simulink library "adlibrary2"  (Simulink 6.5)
undefined symbols (not defined in the file or in its folder): adlibrary2, ADM, DDRII, II, no_bitstream, SRAM, SX, XP, XRC
libraries: xbsIndex_r4 x360, adlibrary2 x9, adlibrary2_d2sram_0 x5, adlibrary2_ddr2dram_1 x4, adlibrary2_ddr_xpi0 x4, adlibrary2_ddr_xpl x3, adlibrary2_xpl32 x1, adlibrary2_xpl64 x1, adlibrary2_zbt64 x1, adlibrary2_zbt4_0 x1, adlibrary2_zbt4_1 x1, adlibrary2_zbt4_2 x1
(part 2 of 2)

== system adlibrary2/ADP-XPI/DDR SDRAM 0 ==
  cache_data_in : Inport
  cache_addr : Inport  Port=2
  cache_write : Inport  Port=3
  ddr_page : Inport  Port=4
  ddr_addr : Inport  Port=5
  ddr_read : Inport  Port=6
  ddr_write : Inport  Port=7
  Assert{1..7,9..10} (9 alike) : xbsIndex_r4/Assert  assert_type=off  type_source=Explicitly  arith_type="Signed  (2's comp)"  n_bits=16  bin_pt=14  assert_rate=on  rate_source=Explicitly  period=ad_get_simulink_period  output_port=on  block_type=assert
  Configurable Subsystem : Subsystem  Tag=configX  BlockChoice=DDR SDRAM 64bit Simulation  mask{memsize=memsize}
      mask prompts: memsize "Simulation Ram Size (Mb)"
  cache_data_out : Outport
  ddr_busy : Outport  Port=2
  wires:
  Assert10/1 -> ddr_busy/1
  Assert9/1 -> cache_data_out/1
  Assert6/1 -> Configurable Subsystem/6(ddr_read)
  Assert5/1 -> Configurable Subsystem/5(ddr_addr)
  Assert4/1 -> Configurable Subsystem/4(ddr_page)
  Assert3/1 -> Configurable Subsystem/3(cache_write)
  Assert2/1 -> Configurable Subsystem/2(cache_addr)
  Assert1/1 -> Configurable Subsystem/1(cache_data_in)
  ddr_write/1 -> Assert7/1
  ddr_read/1 -> Assert6/1
  ddr_addr/1 -> Assert5/1
  ddr_page/1 -> Assert4/1
  cache_write/1 -> Assert3/1
  cache_addr/1 -> Assert2/1
  cache_data_in/1 -> Assert1/1
  Configurable Subsystem/1(cache_data_out) -> Assert9/1
  Configurable Subsystem/2(ddr_busy) -> Assert10/1
  Assert7/1 -> Configurable Subsystem/7(ddr_write)

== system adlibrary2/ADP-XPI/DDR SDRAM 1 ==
  cache_data_in : Inport
  cache_addr : Inport  Port=2
  cache_write : Inport  Port=3
  ddr_page : Inport  Port=4
  ddr_addr : Inport  Port=5
  ddr_read : Inport  Port=6
  ddr_write : Inport  Port=7
  Assert{1..7,9..10} (9 alike) : xbsIndex_r4/Assert  assert_type=off  type_source=Explicitly  arith_type="Signed  (2's comp)"  n_bits=16  bin_pt=14  assert_rate=on  rate_source=Explicitly  period=ad_get_simulink_period  output_port=on  block_type=assert
  Configurable Subsystem : Subsystem  Tag=configX  BlockChoice=DDR SDRAM 64bit Simulation  mask{memsize=memsize}
      mask prompts: memsize "Simulation Ram Size (Mb)"
  cache_data_out : Outport
  ddr_busy : Outport  Port=2
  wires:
  Assert7/1 -> Configurable Subsystem/7(ddr_write)
  Configurable Subsystem/2(ddr_busy) -> Assert10/1
  Configurable Subsystem/1(cache_data_out) -> Assert9/1
  cache_data_in/1 -> Assert1/1
  cache_addr/1 -> Assert2/1
  cache_write/1 -> Assert3/1
  ddr_page/1 -> Assert4/1
  ddr_addr/1 -> Assert5/1
  ddr_read/1 -> Assert6/1
  ddr_write/1 -> Assert7/1
  Assert1/1 -> Configurable Subsystem/1(cache_data_in)
  Assert2/1 -> Configurable Subsystem/2(cache_addr)
  Assert3/1 -> Configurable Subsystem/3(cache_write)
  Assert4/1 -> Configurable Subsystem/4(ddr_page)
  Assert5/1 -> Configurable Subsystem/5(ddr_addr)
  Assert6/1 -> Configurable Subsystem/6(ddr_read)
  Assert9/1 -> cache_data_out/1
  Assert10/1 -> ddr_busy/1

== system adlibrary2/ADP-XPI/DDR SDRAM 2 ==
  cache_data_in : Inport
  cache_addr : Inport  Port=2
  cache_write : Inport  Port=3
  ddr_page : Inport  Port=4
  ddr_addr : Inport  Port=5
  ddr_read : Inport  Port=6
  ddr_write : Inport  Port=7
  Assert{1..7,9..10} (9 alike) : xbsIndex_r4/Assert  assert_type=off  type_source=Explicitly  arith_type="Signed  (2's comp)"  n_bits=16  bin_pt=14  assert_rate=on  rate_source=Explicitly  period=ad_get_simulink_period  output_port=on  block_type=assert
  Configurable Subsystem : Subsystem  Tag=configX  BlockChoice=DDR SDRAM 64bit Simulation  mask{memsize=memsize}
      mask prompts: memsize "Simulation Ram Size (Mb)"
  cache_data_out : Outport
  ddr_busy : Outport  Port=2
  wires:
  Assert10/1 -> ddr_busy/1
  Assert9/1 -> cache_data_out/1
  Assert6/1 -> Configurable Subsystem/6(ddr_read)
  Assert5/1 -> Configurable Subsystem/5(ddr_addr)
  Assert4/1 -> Configurable Subsystem/4(ddr_page)
  Assert3/1 -> Configurable Subsystem/3(cache_write)
  Assert2/1 -> Configurable Subsystem/2(cache_addr)
  Assert1/1 -> Configurable Subsystem/1(cache_data_in)
  ddr_write/1 -> Assert7/1
  ddr_read/1 -> Assert6/1
  ddr_addr/1 -> Assert5/1
  ddr_page/1 -> Assert4/1
  cache_write/1 -> Assert3/1
  cache_addr/1 -> Assert2/1
  cache_data_in/1 -> Assert1/1
  Configurable Subsystem/1(cache_data_out) -> Assert9/1
  Configurable Subsystem/2(ddr_busy) -> Assert10/1
  Assert7/1 -> Configurable Subsystem/7(ddr_write)

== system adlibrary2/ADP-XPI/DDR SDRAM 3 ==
  cache_data_in : Inport
  cache_addr : Inport  Port=2
  cache_write : Inport  Port=3
  ddr_page : Inport  Port=4
  ddr_addr : Inport  Port=5
  ddr_read : Inport  Port=6
  ddr_write : Inport  Port=7
  Assert{1..7,9..10} (9 alike) : xbsIndex_r4/Assert  assert_type=off  type_source=Explicitly  arith_type="Signed  (2's comp)"  n_bits=16  bin_pt=14  assert_rate=on  rate_source=Explicitly  period=ad_get_simulink_period  output_port=on  block_type=assert
  Configurable Subsystem : Subsystem  Tag=configX  BlockChoice=DDR SDRAM 64bit Simulation  mask{memsize=memsize}
      mask prompts: memsize "Simulation Ram Size (Mb)"
  cache_data_out : Outport
  ddr_busy : Outport  Port=2
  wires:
  Assert7/1 -> Configurable Subsystem/7(ddr_write)
  Configurable Subsystem/2(ddr_busy) -> Assert10/1
  Configurable Subsystem/1(cache_data_out) -> Assert9/1
  cache_data_in/1 -> Assert1/1
  cache_addr/1 -> Assert2/1
  cache_write/1 -> Assert3/1
  ddr_page/1 -> Assert4/1
  ddr_addr/1 -> Assert5/1
  ddr_read/1 -> Assert6/1
  ddr_write/1 -> Assert7/1
  Assert1/1 -> Configurable Subsystem/1(cache_data_in)
  Assert2/1 -> Configurable Subsystem/2(cache_addr)
  Assert3/1 -> Configurable Subsystem/3(cache_write)
  Assert4/1 -> Configurable Subsystem/4(ddr_page)
  Assert5/1 -> Configurable Subsystem/5(ddr_addr)
  Assert6/1 -> Configurable Subsystem/6(ddr_read)
  Assert9/1 -> cache_data_out/1
  Assert10/1 -> ddr_busy/1

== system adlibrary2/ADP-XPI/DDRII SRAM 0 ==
  d : Inport
  a : Inport  Port=2
  w : Inport  Port=3
  r : Inport  Port=4
  be : Inport  Port=5
  adlocb_in : Inport  Port=6
  Assert{1..9} (9 alike) : xbsIndex_r4/Assert  assert_type=off  type_source=Explicitly  arith_type="Signed  (2's comp)"  n_bits=16  bin_pt=14  assert_rate=on  rate_source=Explicitly  period=ad_get_simulink_period  output_port=on  block_type=assert
  Configurable Subsystem : Subsystem  Tag=configX  BlockChoice=DDRII SRAM Simulation
  q : Outport
  qv : Outport  Port=2
  adlocb_out : Outport  Port=3
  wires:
  Assert9/1 -> adlocb_out/1
  Assert8/1 -> qv/1
  Assert7/1 -> q/1
  Assert6/1 -> Configurable Subsystem/6(adlocb_in)
  Assert5/1 -> Configurable Subsystem/5(be)
  Assert4/1 -> Configurable Subsystem/4(r)
  Assert3/1 -> Configurable Subsystem/3(w)
  Assert2/1 -> Configurable Subsystem/2(a)
  Assert1/1 -> Configurable Subsystem/1(d)
  Configurable Subsystem/2(qv) -> Assert8/1
  Configurable Subsystem/3(adlocb_out) -> Assert9/1
  adlocb_in/1 -> Assert6/1
  be/1 -> Assert5/1
  r/1 -> Assert4/1
  w/1 -> Assert3/1
  a/1 -> Assert2/1
  d/1 -> Assert1/1
  Configurable Subsystem/1(q) -> Assert7/1

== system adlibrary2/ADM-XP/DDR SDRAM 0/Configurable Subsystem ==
  cache_data_in : Inport
  cache_addr : Inport  Port=2
  cache_write : Inport  Port=3
  ddr_page : Inport  Port=4
  ddr_addr : Inport  Port=5
  ddr_read : Inport  Port=6
  ddr_write : Inport  Port=7
  adlocb_in : Inport  Port=8
  DDR SDRAM 32bit Simulation : adlibrary2_ddr_xpl/DDR SDRAM 32bit Simulation  SystemSampleTime=-1  memsize=memsize
  cache_data_out : Outport
  ddr_busy : Outport  Port=2
  adlocb_out : Outport  Port=3
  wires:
  cache_data_in/1 -> DDR SDRAM 32bit Simulation/1
  cache_addr/1 -> DDR SDRAM 32bit Simulation/2
  cache_write/1 -> DDR SDRAM 32bit Simulation/3
  ddr_page/1 -> DDR SDRAM 32bit Simulation/4
  ddr_addr/1 -> DDR SDRAM 32bit Simulation/5
  ddr_read/1 -> DDR SDRAM 32bit Simulation/6
  ddr_write/1 -> DDR SDRAM 32bit Simulation/7
  adlocb_in/1 -> DDR SDRAM 32bit Simulation/8
  DDR SDRAM 32bit Simulation/1 -> cache_data_out/1
  DDR SDRAM 32bit Simulation/2 -> ddr_busy/1
  DDR SDRAM 32bit Simulation/3 -> adlocb_out/1

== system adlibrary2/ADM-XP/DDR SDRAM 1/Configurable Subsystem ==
  cache_data_in : Inport
  cache_addr : Inport  Port=2
  cache_write : Inport  Port=3
  ddr_page : Inport  Port=4
  ddr_addr : Inport  Port=5
  ddr_read : Inport  Port=6
  ddr_write : Inport  Port=7
  adlocb_in : Inport  Port=8
  DDR SDRAM 32bit Simulation : adlibrary2_ddr_xpl/DDR SDRAM 32bit Simulation  SystemSampleTime=-1  memsize=memsize
  cache_data_out : Outport
  ddr_busy : Outport  Port=2
  adlocb_out : Outport  Port=3
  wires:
  cache_data_in/1 -> DDR SDRAM 32bit Simulation/1
  cache_addr/1 -> DDR SDRAM 32bit Simulation/2
  cache_write/1 -> DDR SDRAM 32bit Simulation/3
  ddr_page/1 -> DDR SDRAM 32bit Simulation/4
  ddr_addr/1 -> DDR SDRAM 32bit Simulation/5
  ddr_read/1 -> DDR SDRAM 32bit Simulation/6
  ddr_write/1 -> DDR SDRAM 32bit Simulation/7
  adlocb_in/1 -> DDR SDRAM 32bit Simulation/8
  DDR SDRAM 32bit Simulation/1 -> cache_data_out/1
  DDR SDRAM 32bit Simulation/2 -> ddr_busy/1
  DDR SDRAM 32bit Simulation/3 -> adlocb_out/1

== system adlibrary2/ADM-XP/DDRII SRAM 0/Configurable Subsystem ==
  d : Inport
  a : Inport  Port=2
  w : Inport  Port=3
  r : Inport  Port=4
  be : Inport  Port=5
  adlocb_in : Inport  Port=6
  DDRII SRAM Simulation : adlibrary2_d2sram_0/DDRII SRAM Simulation  SystemSampleTime=-1
  q : Outport
  qv : Outport  Port=2
  adlocb_out : Outport  Port=3
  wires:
  d/1 -> DDRII SRAM Simulation/1
  a/1 -> DDRII SRAM Simulation/2
  w/1 -> DDRII SRAM Simulation/3
  r/1 -> DDRII SRAM Simulation/4
  be/1 -> DDRII SRAM Simulation/5
  adlocb_in/1 -> DDRII SRAM Simulation/6
  DDRII SRAM Simulation/1 -> q/1
  DDRII SRAM Simulation/2 -> qv/1
  DDRII SRAM Simulation/3 -> adlocb_out/1

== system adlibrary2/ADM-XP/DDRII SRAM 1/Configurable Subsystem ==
  d : Inport
  a : Inport  Port=2
  w : Inport  Port=3
  r : Inport  Port=4
  be : Inport  Port=5
  adlocb_in : Inport  Port=6
  DDRII SRAM Simulation : adlibrary2_d2sram_0/DDRII SRAM Simulation  SystemSampleTime=-1
  q : Outport
  qv : Outport  Port=2
  adlocb_out : Outport  Port=3
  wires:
  d/1 -> DDRII SRAM Simulation/1
  a/1 -> DDRII SRAM Simulation/2
  w/1 -> DDRII SRAM Simulation/3
  r/1 -> DDRII SRAM Simulation/4
  be/1 -> DDRII SRAM Simulation/5
  adlocb_in/1 -> DDRII SRAM Simulation/6
  DDRII SRAM Simulation/1 -> q/1
  DDRII SRAM Simulation/2 -> qv/1
  DDRII SRAM Simulation/3 -> adlocb_out/1

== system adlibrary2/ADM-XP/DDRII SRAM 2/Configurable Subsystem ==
  d : Inport
  a : Inport  Port=2
  w : Inport  Port=3
  r : Inport  Port=4
  be : Inport  Port=5
  adlocb_in : Inport  Port=6
  DDRII SRAM Simulation : adlibrary2_d2sram_0/DDRII SRAM Simulation  SystemSampleTime=-1
  q : Outport
  qv : Outport  Port=2
  adlocb_out : Outport  Port=3
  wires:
  d/1 -> DDRII SRAM Simulation/1
  a/1 -> DDRII SRAM Simulation/2
  w/1 -> DDRII SRAM Simulation/3
  r/1 -> DDRII SRAM Simulation/4
  be/1 -> DDRII SRAM Simulation/5
  adlocb_in/1 -> DDRII SRAM Simulation/6
  DDRII SRAM Simulation/1 -> q/1
  DDRII SRAM Simulation/2 -> qv/1
  DDRII SRAM Simulation/3 -> adlocb_out/1

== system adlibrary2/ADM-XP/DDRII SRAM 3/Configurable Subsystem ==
  d : Inport
  a : Inport  Port=2
  w : Inport  Port=3
  r : Inport  Port=4
  be : Inport  Port=5
  adlocb_in : Inport  Port=6
  DDRII SRAM Simulation : adlibrary2_d2sram_0/DDRII SRAM Simulation  SystemSampleTime=-1
  q : Outport
  qv : Outport  Port=2
  adlocb_out : Outport  Port=3
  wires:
  d/1 -> DDRII SRAM Simulation/1
  a/1 -> DDRII SRAM Simulation/2
  w/1 -> DDRII SRAM Simulation/3
  r/1 -> DDRII SRAM Simulation/4
  be/1 -> DDRII SRAM Simulation/5
  adlocb_in/1 -> DDRII SRAM Simulation/6
  DDRII SRAM Simulation/1 -> q/1
  DDRII SRAM Simulation/2 -> qv/1
  DDRII SRAM Simulation/3 -> adlocb_out/1

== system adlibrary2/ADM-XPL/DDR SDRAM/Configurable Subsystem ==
  cache_data_in : Inport
  cache_addr : Inport  Port=2
  cache_write : Inport  Port=3
  ddr_page : Inport  Port=4
  ddr_addr : Inport  Port=5
  ddr_read : Inport  Port=6
  ddr_write : Inport  Port=7
  adlocb_in : Inport  Port=8
  DDR SDRAM 32bit Simulation : adlibrary2_ddr_xpl/DDR SDRAM 32bit Simulation  SystemSampleTime=-1  memsize=memsize
  cache_data_out : Outport
  ddr_busy : Outport  Port=2
  adlocb_out : Outport  Port=3
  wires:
  cache_data_in/1 -> DDR SDRAM 32bit Simulation/1
  cache_addr/1 -> DDR SDRAM 32bit Simulation/2
  cache_write/1 -> DDR SDRAM 32bit Simulation/3
  ddr_page/1 -> DDR SDRAM 32bit Simulation/4
  ddr_addr/1 -> DDR SDRAM 32bit Simulation/5
  ddr_read/1 -> DDR SDRAM 32bit Simulation/6
  ddr_write/1 -> DDR SDRAM 32bit Simulation/7
  adlocb_in/1 -> DDR SDRAM 32bit Simulation/8
  DDR SDRAM 32bit Simulation/1 -> cache_data_out/1
  DDR SDRAM 32bit Simulation/2 -> ddr_busy/1
  DDR SDRAM 32bit Simulation/3 -> adlocb_out/1

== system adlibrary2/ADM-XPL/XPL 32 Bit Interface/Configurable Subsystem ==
  Data_Read : Inport
  Ack : Inport  Port=2
  Status : Inport  Port=3
  Read IFIFO : Inport  Port=4
  Write OFIFO : Inport  Port=5
  OFIFO_Data : Inport  Port=6
  ADLOCB_IN : Inport  Port=7
  DEBUG_IN : Inport  Port=8
  sstep_clk_sel_default : Inport  Port=9
  XPL 32Bit Simulation : adlibrary2_xpl32/XPL 32Bit Simulation  SystemSampleTime=-1  program=program  clock_ratio=clock_ratio
  Data_Write : Outport
  Addr : Outport  Port=2
  BE : Outport  Port=3
  Write : Outport  Port=4
  Read : Outport  Port=5
  Control : Outport  Port=6
  IFIFO_Data : Outport  Port=7
  IFIFO_Empty : Outport  Port=8
  OFIFO_Full : Outport  Port=9
  ADLOCB_OUT : Outport  Port=10
  DEBUG_OUT : Outport  Port=11
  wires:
  Data_Read/1 -> XPL 32Bit Simulation/1
  Ack/1 -> XPL 32Bit Simulation/2
  Status/1 -> XPL 32Bit Simulation/3
  Read IFIFO/1 -> XPL 32Bit Simulation/4
  Write OFIFO/1 -> XPL 32Bit Simulation/5
  OFIFO_Data/1 -> XPL 32Bit Simulation/6
  ADLOCB_IN/1 -> XPL 32Bit Simulation/7
  DEBUG_IN/1 -> XPL 32Bit Simulation/8
  sstep_clk_sel_default/1 -> XPL 32Bit Simulation/9
  XPL 32Bit Simulation/1 -> Data_Write/1
  XPL 32Bit Simulation/2 -> Addr/1
  XPL 32Bit Simulation/3 -> BE/1
  XPL 32Bit Simulation/4 -> Write/1
  XPL 32Bit Simulation/5 -> Read/1
  XPL 32Bit Simulation/6 -> Control/1
  XPL 32Bit Simulation/7 -> IFIFO_Data/1
  XPL 32Bit Simulation/8 -> IFIFO_Empty/1
  XPL 32Bit Simulation/9 -> OFIFO_Full/1
  XPL 32Bit Simulation/10 -> ADLOCB_OUT/1
  XPL 32Bit Simulation/11 -> DEBUG_OUT/1

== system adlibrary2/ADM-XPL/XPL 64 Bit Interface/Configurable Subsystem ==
  Data_Read : Inport
  Ack : Inport  Port=2
  Status : Inport  Port=3
  Read IFIFO : Inport  Port=4
  Write OFIFO : Inport  Port=5
  OFIFO_Data : Inport  Port=6
  ADLOCB_IN : Inport  Port=7
  DEBUG_IN : Inport  Port=8
  sstep_clk_sel_default : Inport  Port=9
  XPL 64Bit Simulation : adlibrary2_xpl64/XPL 64Bit Simulation  SystemSampleTime=-1  program=program  clock_ratio=clock_ratio
  Data_Write : Outport
  Addr : Outport  Port=2
  BE : Outport  Port=3
  Write : Outport  Port=4
  Read : Outport  Port=5
  Control : Outport  Port=6
  IFIFO_Data : Outport  Port=7
  IFIFO_Empty : Outport  Port=8
  OFIFO_Full : Outport  Port=9
  ADLOCB_OUT : Outport  Port=10
  DEBUG_OUT : Outport  Port=11
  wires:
  Data_Read/1 -> XPL 64Bit Simulation/1
  Ack/1 -> XPL 64Bit Simulation/2
  Status/1 -> XPL 64Bit Simulation/3
  Read IFIFO/1 -> XPL 64Bit Simulation/4
  Write OFIFO/1 -> XPL 64Bit Simulation/5
  OFIFO_Data/1 -> XPL 64Bit Simulation/6
  ADLOCB_IN/1 -> XPL 64Bit Simulation/7
  DEBUG_IN/1 -> XPL 64Bit Simulation/8
  sstep_clk_sel_default/1 -> XPL 64Bit Simulation/9
  XPL 64Bit Simulation/1 -> Data_Write/1
  XPL 64Bit Simulation/2 -> Addr/1
  XPL 64Bit Simulation/3 -> BE/1
  XPL 64Bit Simulation/4 -> Write/1
  XPL 64Bit Simulation/5 -> Read/1
  XPL 64Bit Simulation/6 -> Control/1
  XPL 64Bit Simulation/7 -> IFIFO_Data/1
  XPL 64Bit Simulation/8 -> IFIFO_Empty/1
  XPL 64Bit Simulation/9 -> OFIFO_Full/1
  XPL 64Bit Simulation/10 -> ADLOCB_OUT/1
  XPL 64Bit Simulation/11 -> DEBUG_OUT/1

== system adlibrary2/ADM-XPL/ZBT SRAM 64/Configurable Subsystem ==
  d : Inport
  a : Inport  Port=2
  w : Inport  Port=3
  r : Inport  Port=4
  be : Inport  Port=5
  adlocb_in : Inport  Port=6
  ZBT SRAM 64bit Simulation : adlibrary2_zbt64/ZBT SRAM 64bit Simulation  SystemSampleTime=-1
  q : Outport
  qv : Outport  Port=2
  adlocb_out : Outport  Port=3
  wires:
  d/1 -> ZBT SRAM 64bit Simulation/1
  a/1 -> ZBT SRAM 64bit Simulation/2
  w/1 -> ZBT SRAM 64bit Simulation/3
  r/1 -> ZBT SRAM 64bit Simulation/4
  be/1 -> ZBT SRAM 64bit Simulation/5
  adlocb_in/1 -> ZBT SRAM 64bit Simulation/6
  ZBT SRAM 64bit Simulation/1 -> q/1
  ZBT SRAM 64bit Simulation/2 -> qv/1
  ZBT SRAM 64bit Simulation/3 -> adlocb_out/1

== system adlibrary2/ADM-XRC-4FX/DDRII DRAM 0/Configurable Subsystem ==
  d : Inport
  a : Inport  Port=2
  w : Inport  Port=3
  r : Inport  Port=4
  be : Inport  Port=5
  adlocb_in : Inport  Port=6
  DDRII DRAM Simulation : adlibrary2_ddr2dram_1/DDRII DRAM Simulation  SystemSampleTime=-1
  q : Outport
  qv : Outport  Port=2
  full : Outport  Port=3
  adlocb_out : Outport  Port=4
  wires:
  d/1 -> DDRII DRAM Simulation/1
  a/1 -> DDRII DRAM Simulation/2
  w/1 -> DDRII DRAM Simulation/3
  r/1 -> DDRII DRAM Simulation/4
  be/1 -> DDRII DRAM Simulation/5
  adlocb_in/1 -> DDRII DRAM Simulation/6
  DDRII DRAM Simulation/1 -> q/1
  DDRII DRAM Simulation/2 -> qv/1
  DDRII DRAM Simulation/3 -> full/1
  DDRII DRAM Simulation/4 -> adlocb_out/1

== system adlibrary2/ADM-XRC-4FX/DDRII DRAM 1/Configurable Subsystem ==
  d : Inport
  a : Inport  Port=2
  w : Inport  Port=3
  r : Inport  Port=4
  be : Inport  Port=5
  adlocb_in : Inport  Port=6
  DDRII DRAM Generation : adlibrary2_ddr2dram_1/DDRII DRAM Generation  SystemSampleTime=-1
  q : Outport
  qv : Outport  Port=2
  full : Outport  Port=3
  adlocb_out : Outport  Port=4
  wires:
  d/1 -> DDRII DRAM Generation/1
  a/1 -> DDRII DRAM Generation/2
  w/1 -> DDRII DRAM Generation/3
  r/1 -> DDRII DRAM Generation/4
  be/1 -> DDRII DRAM Generation/5
  adlocb_in/1 -> DDRII DRAM Generation/6
  DDRII DRAM Generation/1 -> q/1
  DDRII DRAM Generation/2 -> qv/1
  DDRII DRAM Generation/3 -> full/1
  DDRII DRAM Generation/4 -> adlocb_out/1

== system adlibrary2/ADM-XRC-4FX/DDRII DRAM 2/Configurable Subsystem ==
  d : Inport
  a : Inport  Port=2
  w : Inport  Port=3
  r : Inport  Port=4
  be : Inport  Port=5
  adlocb_in : Inport  Port=6
  DDRII DRAM Generation : adlibrary2_ddr2dram_1/DDRII DRAM Generation  SystemSampleTime=-1
  q : Outport
  qv : Outport  Port=2
  full : Outport  Port=3
  adlocb_out : Outport  Port=4
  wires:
  d/1 -> DDRII DRAM Generation/1
  a/1 -> DDRII DRAM Generation/2
  w/1 -> DDRII DRAM Generation/3
  r/1 -> DDRII DRAM Generation/4
  be/1 -> DDRII DRAM Generation/5
  adlocb_in/1 -> DDRII DRAM Generation/6
  DDRII DRAM Generation/1 -> q/1
  DDRII DRAM Generation/2 -> qv/1
  DDRII DRAM Generation/3 -> full/1
  DDRII DRAM Generation/4 -> adlocb_out/1

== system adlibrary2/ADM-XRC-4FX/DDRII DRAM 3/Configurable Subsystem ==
  d : Inport
  a : Inport  Port=2
  w : Inport  Port=3
  r : Inport  Port=4
  be : Inport  Port=5
  adlocb_in : Inport  Port=6
  DDRII DRAM Generation : adlibrary2_ddr2dram_1/DDRII DRAM Generation  SystemSampleTime=-1
  q : Outport
  qv : Outport  Port=2
  full : Outport  Port=3
  adlocb_out : Outport  Port=4
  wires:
  d/1 -> DDRII DRAM Generation/1
  a/1 -> DDRII DRAM Generation/2
  w/1 -> DDRII DRAM Generation/3
  r/1 -> DDRII DRAM Generation/4
  be/1 -> DDRII DRAM Generation/5
  adlocb_in/1 -> DDRII DRAM Generation/6
  DDRII DRAM Generation/1 -> q/1
  DDRII DRAM Generation/2 -> qv/1
  DDRII DRAM Generation/3 -> full/1
  DDRII DRAM Generation/4 -> adlocb_out/1

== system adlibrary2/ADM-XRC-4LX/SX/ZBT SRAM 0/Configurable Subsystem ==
  d : Inport
  a : Inport  Port=2
  w : Inport  Port=3
  r : Inport  Port=4
  be : Inport  Port=5
  adlocb_in : Inport  Port=6
  ZBT SRAM 32Bit Simulation : adlibrary2_zbt4_0/ZBT SRAM 32Bit Simulation  SystemSampleTime=-1
  q : Outport
  qv : Outport  Port=2
  adlocb_out : Outport  Port=3
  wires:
  d/1 -> ZBT SRAM 32Bit Simulation/1
  a/1 -> ZBT SRAM 32Bit Simulation/2
  w/1 -> ZBT SRAM 32Bit Simulation/3
  r/1 -> ZBT SRAM 32Bit Simulation/4
  be/1 -> ZBT SRAM 32Bit Simulation/5
  adlocb_in/1 -> ZBT SRAM 32Bit Simulation/6
  ZBT SRAM 32Bit Simulation/1 -> q/1
  ZBT SRAM 32Bit Simulation/2 -> qv/1
  ZBT SRAM 32Bit Simulation/3 -> adlocb_out/1

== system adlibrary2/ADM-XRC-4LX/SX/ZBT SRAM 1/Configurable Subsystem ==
  d : Inport
  a : Inport  Port=2
  w : Inport  Port=3
  r : Inport  Port=4
  be : Inport  Port=5
  adlocb_in : Inport  Port=6
  ZBT SRAM 32Bit Simulation : adlibrary2_zbt4_1/ZBT SRAM 32Bit Simulation  SystemSampleTime=-1
  q : Outport
  qv : Outport  Port=2
  adlocb_out : Outport  Port=3
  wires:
  d/1 -> ZBT SRAM 32Bit Simulation/1
  a/1 -> ZBT SRAM 32Bit Simulation/2
  w/1 -> ZBT SRAM 32Bit Simulation/3
  r/1 -> ZBT SRAM 32Bit Simulation/4
  be/1 -> ZBT SRAM 32Bit Simulation/5
  adlocb_in/1 -> ZBT SRAM 32Bit Simulation/6
  ZBT SRAM 32Bit Simulation/1 -> q/1
  ZBT SRAM 32Bit Simulation/2 -> qv/1
  ZBT SRAM 32Bit Simulation/3 -> adlocb_out/1

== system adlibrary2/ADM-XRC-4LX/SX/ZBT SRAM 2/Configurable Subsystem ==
  d : Inport
  a : Inport  Port=2
  w : Inport  Port=3
  r : Inport  Port=4
  be : Inport  Port=5
  adlocb_in : Inport  Port=6
  ZBT SRAM 32Bit Simulation : adlibrary2_zbt4_2/ZBT SRAM 32Bit Simulation  SystemSampleTime=-1
  q : Outport
  qv : Outport  Port=2
  adlocb_out : Outport  Port=3
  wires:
  d/1 -> ZBT SRAM 32Bit Simulation/1
  a/1 -> ZBT SRAM 32Bit Simulation/2
  w/1 -> ZBT SRAM 32Bit Simulation/3
  r/1 -> ZBT SRAM 32Bit Simulation/4
  be/1 -> ZBT SRAM 32Bit Simulation/5
  adlocb_in/1 -> ZBT SRAM 32Bit Simulation/6
  ZBT SRAM 32Bit Simulation/1 -> q/1
  ZBT SRAM 32Bit Simulation/2 -> qv/1
  ZBT SRAM 32Bit Simulation/3 -> adlocb_out/1

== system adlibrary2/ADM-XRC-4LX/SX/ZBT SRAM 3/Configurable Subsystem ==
  d : Inport
  a : Inport  Port=2
  w : Inport  Port=3
  r : Inport  Port=4
  be : Inport  Port=5
  adlocb_in : Inport  Port=6
  ZBT SRAM 32Bit Simulation : adlibrary2_zbt4_3/ZBT SRAM 32Bit Simulation  SystemSampleTime=-1
  q : Outport
  qv : Outport  Port=2
  adlocb_out : Outport  Port=3
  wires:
  d/1 -> ZBT SRAM 32Bit Simulation/1
  a/1 -> ZBT SRAM 32Bit Simulation/2
  w/1 -> ZBT SRAM 32Bit Simulation/3
  r/1 -> ZBT SRAM 32Bit Simulation/4
  be/1 -> ZBT SRAM 32Bit Simulation/5
  adlocb_in/1 -> ZBT SRAM 32Bit Simulation/6
  ZBT SRAM 32Bit Simulation/1 -> q/1
  ZBT SRAM 32Bit Simulation/2 -> qv/1
  ZBT SRAM 32Bit Simulation/3 -> adlocb_out/1

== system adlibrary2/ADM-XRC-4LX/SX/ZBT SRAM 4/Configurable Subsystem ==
  d : Inport
  a : Inport  Port=2
  w : Inport  Port=3
  r : Inport  Port=4
  be : Inport  Port=5
  adlocb_in : Inport  Port=6
  ZBT SRAM 32Bit Simulation : adlibrary2_zbt4_4/ZBT SRAM 32Bit Simulation  SystemSampleTime=-1
  q : Outport
  qv : Outport  Port=2
  adlocb_out : Outport  Port=3
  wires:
  d/1 -> ZBT SRAM 32Bit Simulation/1
  a/1 -> ZBT SRAM 32Bit Simulation/2
  w/1 -> ZBT SRAM 32Bit Simulation/3
  r/1 -> ZBT SRAM 32Bit Simulation/4
  be/1 -> ZBT SRAM 32Bit Simulation/5
  adlocb_in/1 -> ZBT SRAM 32Bit Simulation/6
  ZBT SRAM 32Bit Simulation/1 -> q/1
  ZBT SRAM 32Bit Simulation/2 -> qv/1
  ZBT SRAM 32Bit Simulation/3 -> adlocb_out/1

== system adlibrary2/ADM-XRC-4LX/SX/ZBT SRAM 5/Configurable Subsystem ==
  d : Inport
  a : Inport  Port=2
  w : Inport  Port=3
  r : Inport  Port=4
  be : Inport  Port=5
  adlocb_in : Inport  Port=6
  ZBT SRAM 32Bit Simulation : adlibrary2_zbt4_5/ZBT SRAM 32Bit Simulation  SystemSampleTime=-1
  q : Outport
  qv : Outport  Port=2
  adlocb_out : Outport  Port=3
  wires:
  d/1 -> ZBT SRAM 32Bit Simulation/1
  a/1 -> ZBT SRAM 32Bit Simulation/2
  w/1 -> ZBT SRAM 32Bit Simulation/3
  r/1 -> ZBT SRAM 32Bit Simulation/4
  be/1 -> ZBT SRAM 32Bit Simulation/5
  adlocb_in/1 -> ZBT SRAM 32Bit Simulation/6
  ZBT SRAM 32Bit Simulation/1 -> q/1
  ZBT SRAM 32Bit Simulation/2 -> qv/1
  ZBT SRAM 32Bit Simulation/3 -> adlocb_out/1

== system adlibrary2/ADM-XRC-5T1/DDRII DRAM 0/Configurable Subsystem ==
  d : Inport
  a : Inport  Port=2
  w : Inport  Port=3
  r : Inport  Port=4
  be : Inport  Port=5
  adlocb_in : Inport  Port=6
  DDRII DRAM Simulation : adlibrary2_ddr2dram5t1_1/DDRII DRAM Simulation  SystemSampleTime=-1
  q : Outport
  qv : Outport  Port=2
  full : Outport  Port=3
  adlocb_out : Outport  Port=4
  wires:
  d/1 -> DDRII DRAM Simulation/1
  a/1 -> DDRII DRAM Simulation/2
  w/1 -> DDRII DRAM Simulation/3
  r/1 -> DDRII DRAM Simulation/4
  be/1 -> DDRII DRAM Simulation/5
  adlocb_in/1 -> DDRII DRAM Simulation/6
  DDRII DRAM Simulation/1 -> q/1
  DDRII DRAM Simulation/2 -> qv/1
  DDRII DRAM Simulation/3 -> full/1
  DDRII DRAM Simulation/4 -> adlocb_out/1

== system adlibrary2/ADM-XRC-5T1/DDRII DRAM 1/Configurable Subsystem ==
  d : Inport
  a : Inport  Port=2
  w : Inport  Port=3
  r : Inport  Port=4
  be : Inport  Port=5
  adlocb_in : Inport  Port=6
  DDRII DRAM Simulation : adlibrary2_ddr2dram5t1_2/DDRII DRAM Simulation  SystemSampleTime=-1
  q : Outport
  qv : Outport  Port=2
  full : Outport  Port=3
  adlocb_out : Outport  Port=4
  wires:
  d/1 -> DDRII DRAM Simulation/1
  a/1 -> DDRII DRAM Simulation/2
  w/1 -> DDRII DRAM Simulation/3
  r/1 -> DDRII DRAM Simulation/4
  be/1 -> DDRII DRAM Simulation/5
  adlocb_in/1 -> DDRII DRAM Simulation/6
  DDRII DRAM Simulation/1 -> q/1
  DDRII DRAM Simulation/2 -> qv/1
  DDRII DRAM Simulation/3 -> full/1
  DDRII DRAM Simulation/4 -> adlocb_out/1

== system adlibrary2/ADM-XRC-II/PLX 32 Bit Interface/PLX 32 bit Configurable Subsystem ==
  Data_Read : Inport
  Ack : Inport  Port=2
  Status : Inport  Port=3
  Read IFIFO : Inport  Port=4
  Write OFIFO : Inport  Port=5
  OFIFO_Data : Inport  Port=6
  ADLOCB_IN : Inport  Port=7
  DEBUG_IN : Inport  Port=8
  sstep_clk_sel_default : Inport  Port=9
  PLX 32Bit Simulation : adlibrary2_plx32/PLX 32Bit Simulation  SystemSampleTime=-1  program=program  clock_ratio=clock_ratio
  Data_Write : Outport
  Addr : Outport  Port=2
  BE : Outport  Port=3
  Write : Outport  Port=4
  Read : Outport  Port=5
  Control : Outport  Port=6
  IFIFO_Data : Outport  Port=7
  IFIFO_Empty : Outport  Port=8
  OFIFO_Full : Outport  Port=9
  ADLOCB_OUT : Outport  Port=10
  DEBUG_OUT : Outport  Port=11
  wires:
  Data_Read/1 -> PLX 32Bit Simulation/1
  Ack/1 -> PLX 32Bit Simulation/2
  Status/1 -> PLX 32Bit Simulation/3
  Read IFIFO/1 -> PLX 32Bit Simulation/4
  Write OFIFO/1 -> PLX 32Bit Simulation/5
  OFIFO_Data/1 -> PLX 32Bit Simulation/6
  ADLOCB_IN/1 -> PLX 32Bit Simulation/7
  DEBUG_IN/1 -> PLX 32Bit Simulation/8
  sstep_clk_sel_default/1 -> PLX 32Bit Simulation/9
  PLX 32Bit Simulation/1 -> Data_Write/1
  PLX 32Bit Simulation/2 -> Addr/1
  PLX 32Bit Simulation/3 -> BE/1
  PLX 32Bit Simulation/4 -> Write/1
  PLX 32Bit Simulation/5 -> Read/1
  PLX 32Bit Simulation/6 -> Control/1
  PLX 32Bit Simulation/7 -> IFIFO_Data/1
  PLX 32Bit Simulation/8 -> IFIFO_Empty/1
  PLX 32Bit Simulation/9 -> OFIFO_Full/1
  PLX 32Bit Simulation/10 -> ADLOCB_OUT/1
  PLX 32Bit Simulation/11 -> DEBUG_OUT/1

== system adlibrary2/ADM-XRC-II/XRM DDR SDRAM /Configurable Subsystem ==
  cache_data_in : Inport
  cache_addr : Inport  Port=2
  cache_write : Inport  Port=3
  ddr_page : Inport  Port=4
  ddr_addr : Inport  Port=5
  ddr_read : Inport  Port=6
  ddr_write : Inport  Port=7
  DDR SDRAM 64bit Simulation : adlibrary2_ddr_xrm/DDR SDRAM 64bit Simulation  SystemSampleTime=-1  memsize=memsize
  cache_data_out : Outport
  ddr_busy : Outport  Port=2
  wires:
  cache_data_in/1 -> DDR SDRAM 64bit Simulation/1
  cache_addr/1 -> DDR SDRAM 64bit Simulation/2
  cache_write/1 -> DDR SDRAM 64bit Simulation/3
  ddr_page/1 -> DDR SDRAM 64bit Simulation/4
  ddr_addr/1 -> DDR SDRAM 64bit Simulation/5
  ddr_read/1 -> DDR SDRAM 64bit Simulation/6
  ddr_write/1 -> DDR SDRAM 64bit Simulation/7
  DDR SDRAM 64bit Simulation/1 -> cache_data_out/1
  DDR SDRAM 64bit Simulation/2 -> ddr_busy/1

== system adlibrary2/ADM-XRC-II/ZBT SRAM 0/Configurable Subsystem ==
  d : Inport
  a : Inport  Port=2
  w : Inport  Port=3
  r : Inport  Port=4
  be : Inport  Port=5
  adlocb_in : Inport  Port=6
  ZBT SRAM 32Bit Simulation : adlibrary2_zbt32_0/ZBT SRAM 32Bit Simulation  SystemSampleTime=-1
  q : Outport
  qv : Outport  Port=2
  adlocb_out : Outport  Port=3
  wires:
  d/1 -> ZBT SRAM 32Bit Simulation/1
  a/1 -> ZBT SRAM 32Bit Simulation/2
  w/1 -> ZBT SRAM 32Bit Simulation/3
  r/1 -> ZBT SRAM 32Bit Simulation/4
  be/1 -> ZBT SRAM 32Bit Simulation/5
  adlocb_in/1 -> ZBT SRAM 32Bit Simulation/6
  ZBT SRAM 32Bit Simulation/1 -> q/1
  ZBT SRAM 32Bit Simulation/2 -> qv/1
  ZBT SRAM 32Bit Simulation/3 -> adlocb_out/1

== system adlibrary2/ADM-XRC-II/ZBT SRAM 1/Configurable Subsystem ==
  d : Inport
  a : Inport  Port=2
  w : Inport  Port=3
  r : Inport  Port=4
  be : Inport  Port=5
  adlocb_in : Inport  Port=6
  ZBT SRAM 32Bit Simulation : adlibrary2_zbt32_1/ZBT SRAM 32Bit Simulation  SystemSampleTime=-1
  q : Outport
  qv : Outport  Port=2
  adlocb_out : Outport  Port=3
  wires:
  d/1 -> ZBT SRAM 32Bit Simulation/1
  a/1 -> ZBT SRAM 32Bit Simulation/2
  w/1 -> ZBT SRAM 32Bit Simulation/3
  r/1 -> ZBT SRAM 32Bit Simulation/4
  be/1 -> ZBT SRAM 32Bit Simulation/5
  adlocb_in/1 -> ZBT SRAM 32Bit Simulation/6
  ZBT SRAM 32Bit Simulation/1 -> q/1
  ZBT SRAM 32Bit Simulation/2 -> qv/1
  ZBT SRAM 32Bit Simulation/3 -> adlocb_out/1

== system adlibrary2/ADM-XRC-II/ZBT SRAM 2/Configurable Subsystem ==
  d : Inport
  a : Inport  Port=2
  w : Inport  Port=3
  r : Inport  Port=4
  be : Inport  Port=5
  adlocb_in : Inport  Port=6
  ZBT SRAM 32Bit Simulation : adlibrary2_zbt32_2/ZBT SRAM 32Bit Simulation  SystemSampleTime=-1
  q : Outport
  qv : Outport  Port=2
  adlocb_out : Outport  Port=3
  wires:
  d/1 -> ZBT SRAM 32Bit Simulation/1
  a/1 -> ZBT SRAM 32Bit Simulation/2
  w/1 -> ZBT SRAM 32Bit Simulation/3
  r/1 -> ZBT SRAM 32Bit Simulation/4
  be/1 -> ZBT SRAM 32Bit Simulation/5
  adlocb_in/1 -> ZBT SRAM 32Bit Simulation/6
  ZBT SRAM 32Bit Simulation/1 -> q/1
  ZBT SRAM 32Bit Simulation/2 -> qv/1
  ZBT SRAM 32Bit Simulation/3 -> adlocb_out/1

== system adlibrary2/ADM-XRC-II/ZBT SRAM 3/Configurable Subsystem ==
  d : Inport
  a : Inport  Port=2
  w : Inport  Port=3
  r : Inport  Port=4
  be : Inport  Port=5
  adlocb_in : Inport  Port=6
  ZBT SRAM 32Bit Simulation : adlibrary2_zbt32_3/ZBT SRAM 32Bit Simulation  SystemSampleTime=-1
  q : Outport
  qv : Outport  Port=2
  adlocb_out : Outport  Port=3
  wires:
  d/1 -> ZBT SRAM 32Bit Simulation/1
  a/1 -> ZBT SRAM 32Bit Simulation/2
  w/1 -> ZBT SRAM 32Bit Simulation/3
  r/1 -> ZBT SRAM 32Bit Simulation/4
  be/1 -> ZBT SRAM 32Bit Simulation/5
  adlocb_in/1 -> ZBT SRAM 32Bit Simulation/6
  ZBT SRAM 32Bit Simulation/1 -> q/1
  ZBT SRAM 32Bit Simulation/2 -> qv/1
  ZBT SRAM 32Bit Simulation/3 -> adlocb_out/1

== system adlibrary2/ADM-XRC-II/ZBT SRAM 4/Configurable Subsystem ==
  d : Inport
  a : Inport  Port=2
  w : Inport  Port=3
  r : Inport  Port=4
  be : Inport  Port=5
  adlocb_in : Inport  Port=6
  ZBT SRAM 32Bit Simulation : adlibrary2_zbt32_4/ZBT SRAM 32Bit Simulation  SystemSampleTime=-1
  q : Outport
  qv : Outport  Port=2
  adlocb_out : Outport  Port=3
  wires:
  d/1 -> ZBT SRAM 32Bit Simulation/1
  a/1 -> ZBT SRAM 32Bit Simulation/2
  w/1 -> ZBT SRAM 32Bit Simulation/3
  r/1 -> ZBT SRAM 32Bit Simulation/4
  be/1 -> ZBT SRAM 32Bit Simulation/5
  adlocb_in/1 -> ZBT SRAM 32Bit Simulation/6
  ZBT SRAM 32Bit Simulation/1 -> q/1
  ZBT SRAM 32Bit Simulation/2 -> qv/1
  ZBT SRAM 32Bit Simulation/3 -> adlocb_out/1

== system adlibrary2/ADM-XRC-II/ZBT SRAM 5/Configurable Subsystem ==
  d : Inport
  a : Inport  Port=2
  w : Inport  Port=3
  r : Inport  Port=4
  be : Inport  Port=5
  adlocb_in : Inport  Port=6
  ZBT SRAM 32Bit Simulation : adlibrary2_zbt32_5/ZBT SRAM 32Bit Simulation  SystemSampleTime=-1
  q : Outport
  qv : Outport  Port=2
  adlocb_out : Outport  Port=3
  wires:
  d/1 -> ZBT SRAM 32Bit Simulation/1
  a/1 -> ZBT SRAM 32Bit Simulation/2
  w/1 -> ZBT SRAM 32Bit Simulation/3
  r/1 -> ZBT SRAM 32Bit Simulation/4
  be/1 -> ZBT SRAM 32Bit Simulation/5
  adlocb_in/1 -> ZBT SRAM 32Bit Simulation/6
  ZBT SRAM 32Bit Simulation/1 -> q/1
  ZBT SRAM 32Bit Simulation/2 -> qv/1
  ZBT SRAM 32Bit Simulation/3 -> adlocb_out/1

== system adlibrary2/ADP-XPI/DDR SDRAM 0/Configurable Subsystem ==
  cache_data_in : Inport
  cache_addr : Inport  Port=2
  cache_write : Inport  Port=3
  ddr_page : Inport  Port=4
  ddr_addr : Inport  Port=5
  ddr_read : Inport  Port=6
  ddr_write : Inport  Port=7
  DDR SDRAM 64bit Simulation : adlibrary2_ddr_xpi0/DDR SDRAM 64bit Simulation  SystemSampleTime=-1  memsize=memsize
  cache_data_out : Outport
  ddr_busy : Outport  Port=2
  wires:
  cache_data_in/1 -> DDR SDRAM 64bit Simulation/1
  cache_addr/1 -> DDR SDRAM 64bit Simulation/2
  cache_write/1 -> DDR SDRAM 64bit Simulation/3
  ddr_page/1 -> DDR SDRAM 64bit Simulation/4
  ddr_addr/1 -> DDR SDRAM 64bit Simulation/5
  ddr_read/1 -> DDR SDRAM 64bit Simulation/6
  ddr_write/1 -> DDR SDRAM 64bit Simulation/7
  DDR SDRAM 64bit Simulation/1 -> cache_data_out/1
  DDR SDRAM 64bit Simulation/2 -> ddr_busy/1

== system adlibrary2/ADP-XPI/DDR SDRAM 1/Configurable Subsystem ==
  cache_data_in : Inport
  cache_addr : Inport  Port=2
  cache_write : Inport  Port=3
  ddr_page : Inport  Port=4
  ddr_addr : Inport  Port=5
  ddr_read : Inport  Port=6
  ddr_write : Inport  Port=7
  DDR SDRAM 64bit Simulation : adlibrary2_ddr_xpi0/DDR SDRAM 64bit Simulation  SystemSampleTime=-1  memsize=memsize
  cache_data_out : Outport
  ddr_busy : Outport  Port=2
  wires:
  cache_data_in/1 -> DDR SDRAM 64bit Simulation/1
  cache_addr/1 -> DDR SDRAM 64bit Simulation/2
  cache_write/1 -> DDR SDRAM 64bit Simulation/3
  ddr_page/1 -> DDR SDRAM 64bit Simulation/4
  ddr_addr/1 -> DDR SDRAM 64bit Simulation/5
  ddr_read/1 -> DDR SDRAM 64bit Simulation/6
  ddr_write/1 -> DDR SDRAM 64bit Simulation/7
  DDR SDRAM 64bit Simulation/1 -> cache_data_out/1
  DDR SDRAM 64bit Simulation/2 -> ddr_busy/1

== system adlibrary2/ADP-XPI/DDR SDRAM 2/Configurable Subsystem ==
  cache_data_in : Inport
  cache_addr : Inport  Port=2
  cache_write : Inport  Port=3
  ddr_page : Inport  Port=4
  ddr_addr : Inport  Port=5
  ddr_read : Inport  Port=6
  ddr_write : Inport  Port=7
  DDR SDRAM 64bit Simulation : adlibrary2_ddr_xpi0/DDR SDRAM 64bit Simulation  SystemSampleTime=-1  memsize=memsize
  cache_data_out : Outport
  ddr_busy : Outport  Port=2
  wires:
  cache_data_in/1 -> DDR SDRAM 64bit Simulation/1
  cache_addr/1 -> DDR SDRAM 64bit Simulation/2
  cache_write/1 -> DDR SDRAM 64bit Simulation/3
  ddr_page/1 -> DDR SDRAM 64bit Simulation/4
  ddr_addr/1 -> DDR SDRAM 64bit Simulation/5
  ddr_read/1 -> DDR SDRAM 64bit Simulation/6
  ddr_write/1 -> DDR SDRAM 64bit Simulation/7
  DDR SDRAM 64bit Simulation/1 -> cache_data_out/1
  DDR SDRAM 64bit Simulation/2 -> ddr_busy/1

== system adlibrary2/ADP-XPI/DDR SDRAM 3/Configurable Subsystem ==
  cache_data_in : Inport
  cache_addr : Inport  Port=2
  cache_write : Inport  Port=3
  ddr_page : Inport  Port=4
  ddr_addr : Inport  Port=5
  ddr_read : Inport  Port=6
  ddr_write : Inport  Port=7
  DDR SDRAM 64bit Simulation : adlibrary2_ddr_xpi0/DDR SDRAM 64bit Simulation  SystemSampleTime=-1  memsize=memsize
  cache_data_out : Outport
  ddr_busy : Outport  Port=2
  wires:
  cache_data_in/1 -> DDR SDRAM 64bit Simulation/1
  cache_addr/1 -> DDR SDRAM 64bit Simulation/2
  cache_write/1 -> DDR SDRAM 64bit Simulation/3
  ddr_page/1 -> DDR SDRAM 64bit Simulation/4
  ddr_addr/1 -> DDR SDRAM 64bit Simulation/5
  ddr_read/1 -> DDR SDRAM 64bit Simulation/6
  ddr_write/1 -> DDR SDRAM 64bit Simulation/7
  DDR SDRAM 64bit Simulation/1 -> cache_data_out/1
  DDR SDRAM 64bit Simulation/2 -> ddr_busy/1

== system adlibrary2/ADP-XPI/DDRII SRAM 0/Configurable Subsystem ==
  d : Inport
  a : Inport  Port=2
  w : Inport  Port=3
  r : Inport  Port=4
  be : Inport  Port=5
  adlocb_in : Inport  Port=6
  DDRII SRAM Simulation : adlibrary2_d2sram_0/DDRII SRAM Simulation  SystemSampleTime=-1
  q : Outport
  qv : Outport  Port=2
  adlocb_out : Outport  Port=3
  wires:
  d/1 -> DDRII SRAM Simulation/1
  a/1 -> DDRII SRAM Simulation/2
  w/1 -> DDRII SRAM Simulation/3
  r/1 -> DDRII SRAM Simulation/4
  be/1 -> DDRII SRAM Simulation/5
  adlocb_in/1 -> DDRII SRAM Simulation/6
  DDRII SRAM Simulation/1 -> q/1
  DDRII SRAM Simulation/2 -> qv/1
  DDRII SRAM Simulation/3 -> adlocb_out/1
